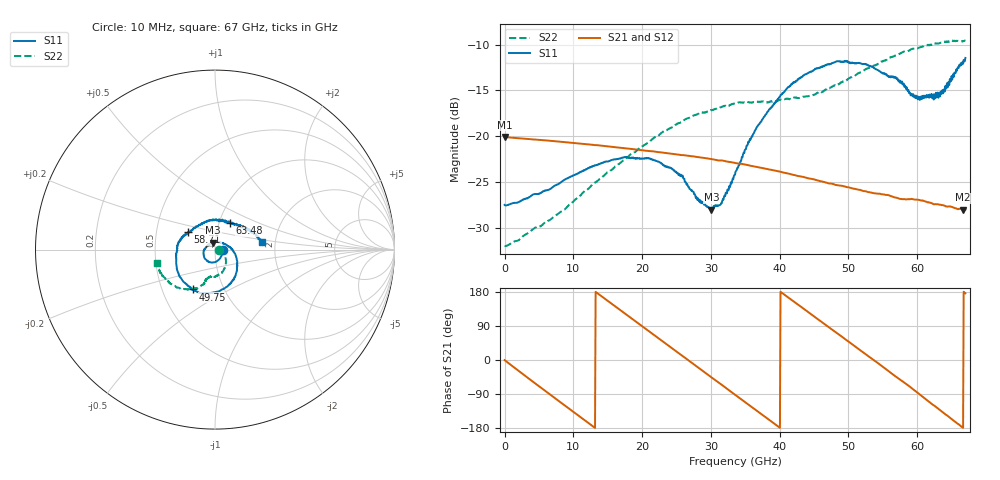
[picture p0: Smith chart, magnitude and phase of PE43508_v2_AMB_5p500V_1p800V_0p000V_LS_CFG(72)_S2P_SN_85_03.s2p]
!Keysight Technologies,N5227A,US51270237,A.10.43.00
!Date: Wednesday, August 22, 2018 17:14:08
!Correction: S11(Full 2 Port(1,3))
!S31(Full 2 Port(1,3))
!S13(Full 2 Port(1,3))
!S33(Full 2 Port(1,3))
!S2P File: Measurements: S11, S31, S13, S33:
# Hz S  dB  R 50
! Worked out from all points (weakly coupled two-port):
!   801 points, 10 MHz to 67 GHz, reference 50 ohm
!   highest |S21| = -20.10 dB at 10 MHz (marker M1); lowest = -28.0 dB at 66.67 GHz (marker M2)
!   lowest |S11| = -28.1 dB at 30.07 GHz (marker M3), VSWR 1.08, Z = 48.8 + j3.72 ohm
!   |S11| at or under -10 dB: start of sweep to end of sweep
!   |S22| runs from -32.0 to -9.6 dB; largest |S21 - S12| = 0.00051
!   S11 on the Smith chart (normalised r, x): 10 MHz: 1.09, -0.00; 49.75 GHz: 0.71, -0.34; 58.71 GHz: 0.73, +0.15; 63.48 GHz: 1.13, +0.34; 67 GHz: 1.71, +0.15
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1e7  -27.52 -0.7  -20.10 -0.2  -20.10 -0.2  -32.02 -0.5
5.787888e9  -26.00 -42.2  -20.46 -79.8  -20.47 -79.8  -29.50 -6.7
1.123082e10  -23.84 -77.6  -20.84 -153.4  -20.84 -153.3  -26.31 -20.9
1.759488e10  -22.30 -115.6  -21.34 121.3  -21.34 121.3  -22.50 -38.7
2.236791e10  -22.80 -147.9  -21.76 57.4  -21.75 57.4  -19.95 -53.8
2.571741e10  -24.36 -179.5  -22.08 12.8  -22.07 12.8  -18.50 -64.7
2.81458e10  -26.81 145.6  -22.30 -19.7  -22.31 -19.8  -17.56 -72.6
3.007176e10  -28.05 105.9  -22.51 -45.7  -22.51 -45.7  -17.19 -78.9
3.14953e10  -27.33 70.6  -22.66 -64.4  -22.66 -64.4  -16.86 -83.7
3.3505e10  -24.22 30.3  -22.94 -91.6  -22.94 -91.7  -16.45 -89.7
3.55147e10  -20.69 1.9  -23.20 -118.5  -23.21 -118.5  -16.29 -94.0
3.836178e10  -17.26 -26.6  -23.64 -156.4  -23.65 -156.4  -16.31 -99.8
4.137632e10  -14.62 -52.8  -24.12 163.2  -24.12 163.3  -15.98 -102.9
4.472582e10  -12.92 -80.3  -24.69 118.7  -24.68 118.8  -15.56 -105.3
4.975008e10  -11.88 -119.3  -25.58 52.0  -25.56 52.0  -13.90 -108.6
5.276462e10  -12.26 -145.7  -26.09 11.6  -26.08 11.5  -12.61 -114.4
5.586291e10  -13.56 -178.5  -26.46 -30.1  -26.45 -30.4  -11.48 -123.7
5.870999e10  -14.95 147.3  -26.90 -67.5  -26.90 -67.7  -10.68 -133.1
6.130585e10  -15.80 101.8  -27.18 -104.5  -27.18 -104.9  -10.09 -143.2
6.348302e10  -15.38 59.9  -27.53 -134.6  -27.57 -135.2  -9.78 -152.1
6.666505e10  -12.10 13.8  -28.04 -179.0  -28.11 -179.0  -9.61 -164.9
6.7e10  -11.46 8.7  -28.03 176.0  -28.12 176.0  -9.57 -166.7
